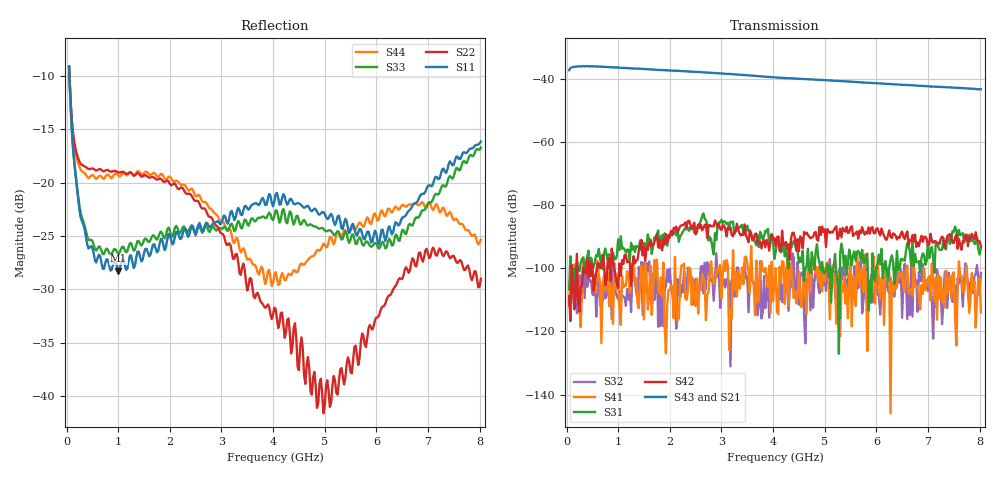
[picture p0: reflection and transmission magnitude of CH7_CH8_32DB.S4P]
!Agilent Technologies,E5071C,MY46316741,A.11.02
!Date: Mon Jun 01 10:28:04 2026
!Data & Calibration Information:
!1:CH7 INPUT 2:CH7 OUTPUT 3:CH8 INPUT 4:CH8 OUTPUT
!Freq	S11:SOLT4(ON)	S12:SOLT4(ON)	S13:SOLT4(ON)	S14:SOLT4(ON)
!	S21:SOLT4(ON)	S22:SOLT4(ON)	S23:SOLT4(ON)	S24:SOLT4(ON)
!	S31:SOLT4(ON)	S32:SOLT4(ON)	S33:SOLT4(ON)	S34:SOLT4(ON)
!	S41:SOLT4(ON)	S42:SOLT4(ON)	S43:SOLT4(ON)	S44:SOLT4(ON)
!PortZ  Port1:50+j0  Port2:50+j0  Port3:50+j0  Port4:50+j0
!Above PortZ is port z conversion or system Z0 setting when saving the data.
!When reading, reference impedance value at option line is always used.
# Hz S dB R 50
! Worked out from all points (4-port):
!   320 points, 50 MHz to 8.025 GHz, reference 50 ohm
!   strongest paths, dB at 50 MHz, 2.05 GHz, 4.05 GHz, 6.05 GHz, 8.025 GHz:
!     S43: -37.3, -37.5, -39.6, -41.5, -43.4
!     S21: -37.5, -37.6, -39.8, -41.7, -43.6
!     S42: -108.8, -89.6, -92.9, -88.8, -93.0
!     S31: -106.7, -89.0, -94.8, -95.7, -93.6
!     S41: -111.8, -105.8, -99.9, -103.3, -114.0
!     S32: -110.8, -108.2, -106.0, -108.3, -101.5
!   lowest |S11| = -28.3 dB at 1 GHz (marker M1), VSWR 1.08, Z = 47.7 - j3.01 ohm
!   |S11| at or under -10 dB: 57.22 MHz to end of sweep
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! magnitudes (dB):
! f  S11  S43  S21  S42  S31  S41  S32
! 50 MHz  -9.1  -37.3  -37.5  -108.8  -106.7  -111.8  -110.8
! 275 MHz  -23.3  -36.1  -36.2  -105.6  -98.3  -118.6  -116.3
! 1 GHz  -28.3  -36.5  -36.6  -106.3  -90.8  -104.4  -109.9
! 2.675 GHz  -24.1  -38.1  -38.2  -86.3  -84.3  -105.0  -98.3
! 4.975 GHz  -22.7  -40.5  -40.7  -88.5  -101.4  -99.8  -105.2
! 6.7 GHz  -22.1  -42.1  -42.4  -89.5  -90.6  -108.6  -115.3
! 8.025 GHz  -16.1  -43.4  -43.6  -93.0  -93.6  -114.0  -101.5
